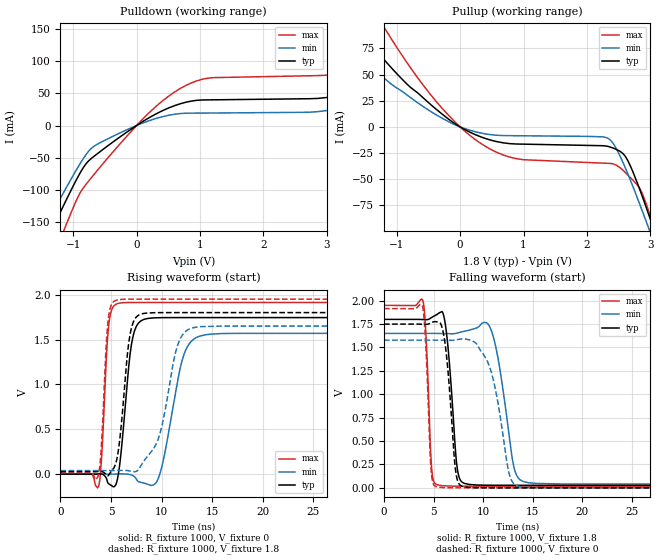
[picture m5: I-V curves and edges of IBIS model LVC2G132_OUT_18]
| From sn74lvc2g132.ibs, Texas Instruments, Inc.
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[Model]   LVC2G132_OUT_18
Model_type  Output
Vref =   0
Rref =   1000
Cref =   30p
Vmeas =   0.9
| variable   typ   min   max
C_comp   9.96pF   6.41pF   16.10pF
| C_pullup   9.16pF   6.41pF   10.37pF
| C_pulldown   10.75pF   6.91pF   16.10pF
[Temperature Range]   40   100   -40
| Ambient temperature   25   85   -40
[Voltage range]   1.8   1.65   1.95
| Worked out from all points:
|   slope of the pulldown table from 0 to 0.27 V, typ, clamps not added: 16.8 ohm
|   slope of the pullup table from 0 to 0.27 V, typ, clamps not added: 33 ohm
|   rising waveform, R_fixture 1000, V_fixture 0: 20-80 % time 867ps typ, 1.55ns min, 507ps max; typ from 0 V to 1.74 V
|   falling waveform, R_fixture 1000, V_fixture 1.8: 20-80 % time 716ps typ, 1.28ns min, 429ps max; typ from 1.8 V to 0.027 V
|   rising waveform, R_fixture 1000, V_fixture 1.8: 20-80 % time 875ps typ, 1.76ns min, 506ps max; typ from 0.027 V to 1.8 V
|   falling waveform, R_fixture 1000, V_fixture 0: 20-80 % time 750ps typ, 1.59ns min, 435ps max; typ from 1.75 V to 0 V
[Pulldown]
| LVC2G132_OUT_18
|   Voltage   I(typ)   I(min)   I(max)
-5.5V     -1.02A     -914.2mA   -1.211A
-1.49V    -194.3mA   -166.1mA   -248.7mA
-1.27V    -148.7mA   -125.7mA   -193.7mA
-1.11V    -116mA     -96.9mA    -154.1mA
-645mV    -45.9mA    -30.54mA   -72.92mA
690mV     33.84mA    18.58mA    57.6mA
3.205V    47.35mA    26.83mA    81.75mA
4.215V    79.09mA    21.52mA    130mA
4.445V    47.14mA    21.65mA    144.9mA
4.62V     44.43mA    21.75mA    152.8mA
5.01V     44.71mA    21.98mA    83.26mA
11V       50.71mA    25.31mA    93.17mA
[Pullup]
| LVC2G132_OUT_18
|   Voltage   I(typ)   I(min)   I(max)
-5.5V     449.7mA    254mA      638.5mA
-2.225V   143.3mA    107.6mA    207.3mA
-1.755V   105.1mA    78.04mA    153.5mA
-1.195V   63.95mA    46.44mA    94.81mA
-375mV    16.75mA    11.48mA    24.15mA
420mV     -11.47mA   -6.842mA   -19.31mA
2.34V     -18.75mA   -11.19mA   -34.79mA
2.61V     -28.71mA   -39.94mA   -43.87mA
2.825V    -58.63mA   -72.76mA   -58mA
2.97V     -83.15mA   -96.31mA   -80.03mA
3.12V     -109.8mA   -121.4mA   -108.9mA
11V       -1.703A    -1.583A    -1.935A
[Ramp]
| LVC2G132_OUT_18
| variable   typ   min   max
dV/dt_r   1.13/9.36E-10   1.02/1.67E-09   1.24/5.46E-10
dV/dt_f   1.11/7.64E-10   1.04/1.41E-09   1.20/4.54E-10
R_load = 1000
[Rising Waveform]
| LVC2G132_OUT_18
R_fixture =   1000
C_fixture =   0
L_fixture =   0
V_fixture =   0
V_fixture_min = 0
V_fixture_max = 0
|   Time   V(typ)   V(min)   V(max)
0s        114pV      8.171nV    2.621nV
3.765ns   2.376mV    518.6nV    -137.5mV
4.76ns    -105.6mV   -136.5uV   1.641V
5.63ns    -59.3mV    1.378mV    1.899V
7.025ns   1.445V     -10.14mV   1.913V
8.235ns   1.723V     -97.83mV   1.913V
9.715ns   1.743V     -36.45mV   1.913V
12.06ns   1.744V     1.277V     1.913V
13.73ns   1.744V     1.536V     1.913V
50ns      1.744V     1.569V     1.913V
[Falling Waveform]
| LVC2G132_OUT_18
R_fixture =   1000
C_fixture =   0
L_fixture =   0
V_fixture =   1.8
V_fixture_min = 1.65
V_fixture_max = 1.95
|   Time   V(typ)   V(min)   V(max)
0s        1.8V       1.65V      1.95V
3.945ns   1.798V     1.65V      1.992V
4.785ns   1.819V     1.65V      237.3mV
5.315ns   1.851V     1.65V      35.07mV
6.16ns    1.767V     1.648V     21.1mV
7.34ns    249.4mV    1.653V     18.58mV
8.09ns    48.38mV    1.673V     18.33mV
10.8ns    28.03mV    1.691V     18.21mV
14.04ns   27.33mV    67.75mV    18.21mV
50ns      27.28mV    39.55mV    18.2mV
[Rising Waveform]
| LVC2G132_OUT_18
R_fixture =   1000
C_fixture =   0
L_fixture =   0
V_fixture =   1.8
V_fixture_min = 1.65
V_fixture_max = 1.95
|   Time   V(typ)   V(min)   V(max)
0s        27.26mV    39.51mV    18.19mV
3.725ns   29.23mV    39.51mV    -20.64mV
4.03ns    29.45mV    39.51mV    284.4mV
4.695ns   -18.34mV   39.4mV     1.691V
5.5ns     131.9mV    40.12mV    1.937V
6.855ns   1.536V     35.66mV    1.95V
7.96ns    1.783V     94.76mV    1.95V
9.65ns    1.799V     385.2mV    1.95V
12.93ns   1.8V       1.625V     1.95V
50ns      1.8V       1.65V      1.95V
[Falling Waveform]
| LVC2G132_OUT_18
R_fixture =   1000
C_fixture =   0
L_fixture =   0
V_fixture =   0
V_fixture_min = 0
V_fixture_max = 0
|   Time   V(typ)   V(min)   V(max)
0s        1.749V     1.578V     1.916V
3.88ns    1.748V     1.578V     1.94V
4.735ns   1.764V     1.578V     215.7mV
5.22ns    1.776V     1.578V     14.57mV
6.075ns   1.604V     1.577V     2.189mV
7.2ns     203.5mV    1.579V     290.5uV
7.89ns    16.47mV    1.591V     103.8uV
10.61ns   372.8uV    1.306V     18.67uV
13.47ns   47.89uV    19.13mV    16.08uV
50ns      15.9uV     34.32uV    7.773uV
